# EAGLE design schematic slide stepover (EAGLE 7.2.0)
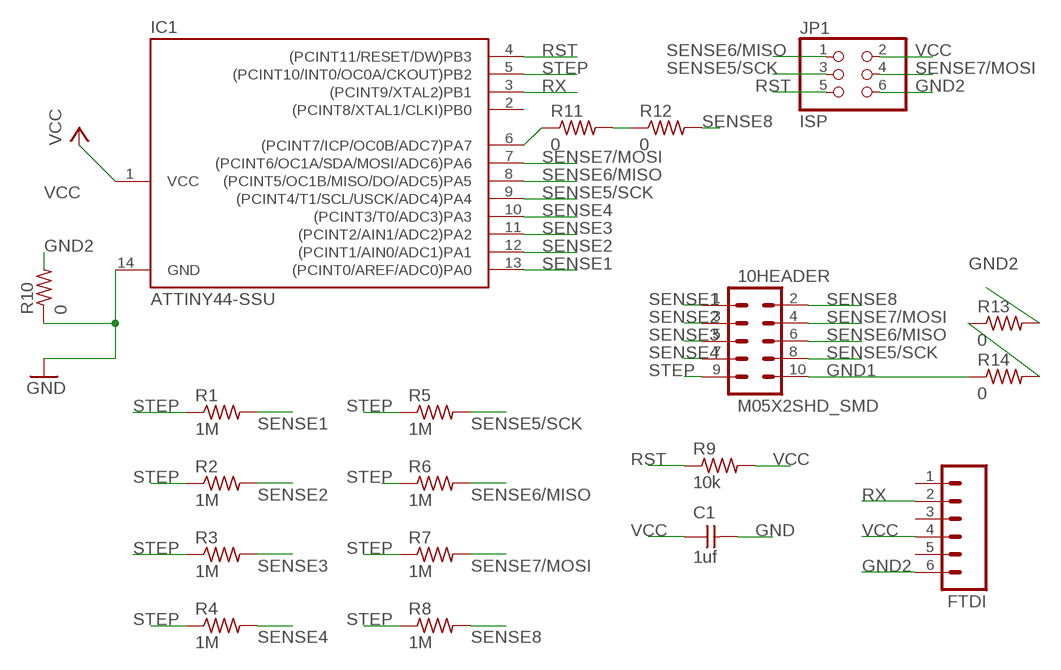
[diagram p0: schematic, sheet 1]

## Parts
10HEADER  M05X2SHD_SMD  [2X5-SHROUDED_SMD]
C1  1uf  UNPOLARIZED_CAPACITOR1206  [1206]
FTDI  M06SMD  [1X06-SMD]
IC1  ATTINY44-SSU  [SOIC14]
JP1  ISP  PINHD-2X3-SMD  [2X03SMD]
R1  1M  RESISTOR1206  [1206]
R2  1M  RESISTOR1206  [1206]
R3  1M  RESISTOR1206  [1206]
R4  1M  RESISTOR1206  [1206]
R5  1M  RESISTOR1206  [1206]
R6  1M  RESISTOR1206  [1206]
R7  1M  RESISTOR1206  [1206]
R8  1M  RESISTOR1206  [1206]
R9  10k  RESISTOR1206  [1206]
R10  0  RESISTOR1206  [1206]
R11  0  RESISTOR1206  [1206]
R12  0  RESISTOR1206  [1206]
R13  0  RESISTOR1206  [1206]
R14  0  RESISTOR1206  [1206]

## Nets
GND: C1.2 IC1.14(GND) R10.1
GND1: 10HEADER.10 R14.1
GND2: FTDI.6 JP1.6 R10.2 R13.2
N$1: R11.2 R12.1
N$2: R13.1 R14.2
N$3: IC1.6((PCINT7/ICP/OC0B/ADC7)PA7) R11.1
RST: IC1.4((PCINT11/RESET/DW)PB3) JP1.5 R9.1
RX: FTDI.2 IC1.3((PCINT9/XTAL2)PB1)
SENSE1: 10HEADER.1 IC1.13((PCINT0/AREF/ADC0)PA0) R1.2
SENSE2: 10HEADER.3 IC1.12((PCINT1/AIN0/ADC1)PA1) R2.2
SENSE3: 10HEADER.5 IC1.11((PCINT2/AIN1/ADC2)PA2) R3.2
SENSE4: 10HEADER.7 IC1.10((PCINT3/T0/ADC3)PA3) R4.2
SENSE5/SCK: 10HEADER.8 IC1.9((PCINT4/T1/SCL/USCK/ADC4)PA4) JP1.3 R5.2
SENSE6/MISO: 10HEADER.6 IC1.8((PCINT5/OC1B/MISO/DO/ADC5)PA5) JP1.1 R6.2
SENSE7/MOSI: 10HEADER.4 IC1.7((PCINT6/OC1A/SDA/MOSI/ADC6)PA6) JP1.4 R7.2
SENSE8: 10HEADER.2 R8.2 R12.2
STEP: 10HEADER.9 IC1.5((PCINT10/INT0/OC0A/CKOUT)PB2) R1.1 R2.1 R3.1 R4.1 R5.1 R6.1 R7.1 R8.1
VCC: C1.1 FTDI.4 IC1.1(VCC) JP1.2 R9.2
Unconnected: FTDI.1 FTDI.3 FTDI.5 IC1.2((PCINT8/XTAL1/CLKI)PB0)

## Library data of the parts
10HEADER = 01_SparkFun:M05X2: Header 5x2 Standard 10-pin dual row 0.1" header. Commonly used with AVR-ISP. Use with Spark Fun Electronics SKU: PRT-00778
C1 = 01_ng:UNPOLARIZED_CAPACITOR: unpolarized_capacitor
FTDI = 01_SparkFun:M06: Header 6 Standard 6-pin 0.1" header. Use with straight break away headers (SKU : PRT-00116), right angle break away headers (PRT-00553), swiss pins (PRT-00743), machine pins (PRT-00117), and female headers (PRT-00115). Molex polarized connector foot print use with SKU : PRT-08094 with associated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
IC1 = 01_fab:ATTINY44
JP1 = 01_fab:PINHD-2X3-SMD: PIN HEADER
R1-R14 = 01_ng:RESISTOR

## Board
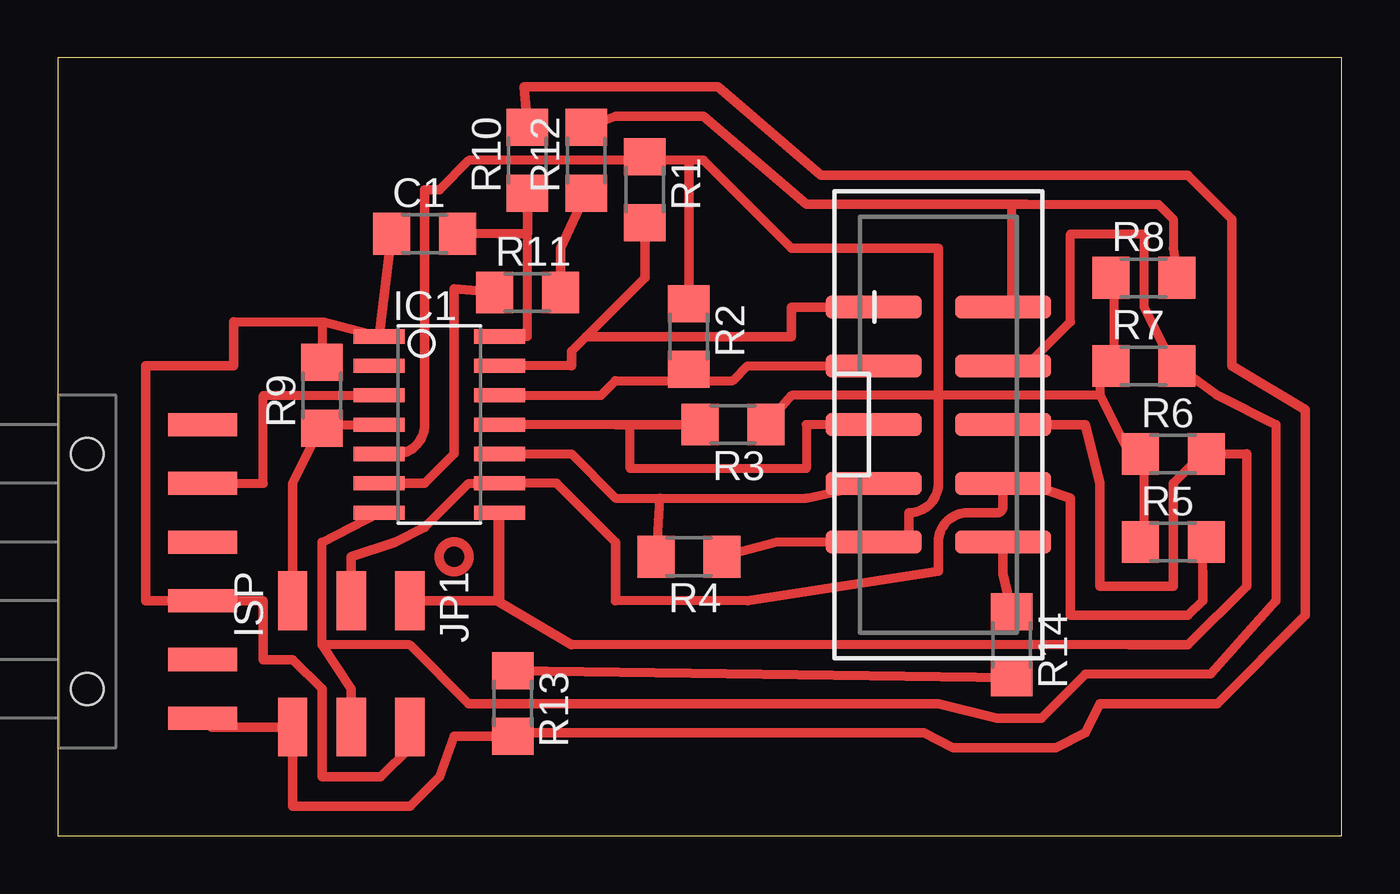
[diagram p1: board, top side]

Size 55.55 x 33.64 mm. Coordinates in mm from the lower left corner, seen from the top.
Outline: 0,0 55.55,0 55.55,33.64 0,33.64 0,0
Copper layers (1*16): Top 0.035mm / dielectric 1.5mm / Bottom 0.035mm
Design rules "default *": minimum track width 0.4mm, minimum drill 0.8mm, track to track 0.4mm, track to pad 0.4mm, pad to pad 0.4mm, via to via 0.4mm, smd to smd 8mil, copper to edge 0mil, drill to drill 0.8mm, minimum pad ring 10mil, minimum via ring 8mil, stop-mask expansion 4mil, vias tented up to drill 0mil, thermal gap 10mil

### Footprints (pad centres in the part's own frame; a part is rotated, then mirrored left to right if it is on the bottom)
2X5-SHROUDED_SMD = smd 4.15 x 1: 1 -2.794,5.08; 2 2.794,5.08; 3 -2.794,2.54; 4 2.794,2.54; 5 -2.794,0; 6 2.794,0; 7 -2.794,-2.54; 8 2.794,-2.54; 9 -2.794,-5.08; 10 2.794,-5.08
1206 = smd 1.6 x 1.803: 1 -1.422,0; 2 1.422,0
1X06-SMD = smd 1 x 3: 1 -6.35,5; 2 -3.81,5; 3 -1.27,5; 4 1.27,5; 5 3.81,5; 6 6.35,5 | hole 1.4: -5.08,0; 5.08,0
SOIC14 = smd 0.61 x 2.21: 1 -3.81,-2.603; 2 -2.54,-2.603; 3 -1.27,-2.603; 4 0,-2.603; 5 1.27,-2.603; 6 2.54,-2.603; 7 3.81,-2.603; 8 3.81,2.603; 9 2.54,2.603; 10 1.27,2.603; 11 0,2.603; 12 -1.27,2.603; 13 -2.54,2.603; 14 -3.81,2.603
2X03SMD = smd 2.54 x 1.27: 1 -2.54,2.54; 2 2.92,2.54; 3 -2.54,0; 4 2.92,0; 5 -2.54,-2.54; 6 2.92,-2.54

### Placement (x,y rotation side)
10HEADER  38.1,17.78 0 top
C1  15.88,26.04 0 top
FTDI  1.27,11.43 270 top
IC1  16.51,17.78 270 top
JP1  12.7,7.62 270 top
R1  25.4,27.94 270 top
R2  27.3,21.59 270 top
R3  29.21,17.78 180 top
R4  27.3,12.07 180 top
R5  48.26,12.7 0 top
R6  48.26,16.51 0 top
R7  46.99,20.32 0 top
R8  46.99,24.13 0 top
R9  11.43,19.05 90 top
R10  20.32,29.21 90 top
R11  20.32,23.5 0 top
R12  22.86,29.21 90 top
R13  19.68,5.71 270 top
R14  41.27,8.26 270 top

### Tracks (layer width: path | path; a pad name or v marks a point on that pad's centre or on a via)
GND
  Top 0.4: 20.32,26.04 20.32,21.59 IC1.14 | 19.05,26.04 C1.2
  Top 0.406: 19.05,26.04 20.32,26.04 R10.1
GND1
  Top 0.406: 10HEADER.10 40.89,11.33 R14.1
GND2
  Top 0.406: FTDI.6 6.65,4.7 JP1.6 10.16,1.27 15.24,1.27 16.51,2.54 17.14,4.29 R13.2 20.32,4.45 37.46,4.45 38.73,3.81 43.18,3.81 44.45,4.45 45.08,5.71 50.16,5.71 53.97,9.53 53.97,18.41 50.8,20.32 50.8,26.67 48.89,28.57 33.02,28.57 28.57,32.38 20.17,32.38 R10.2
N$1
  Top 0.406: R11.2 21.74,25.4 R12.1
N$2
  Top 0.406: R13.1 R14.2
N$3
  Top 0.406: R11.1 17.14,23.65 17.14,16.51 15.88,15.24 IC1.6
RST
  Top 0.4: 10.16,15.24 11.43,17.78 | 11.43,17.78 R9.1 | 11.43,17.78 IC1.4
  Top 0.406: 10.16,15.24 JP1.5
RX
  Top 0.4: IC1.3 8.89,19.05 8.89,15.24 FTDI.2
SENSE1
  Top 0.4: 34.92,22.86 10HEADER.1 | 22.23,20.32 IC1.13 | 25.4,26.67 R1.2
  Top 0.406: 22.86,21.59 31.75,21.59 31.75,22.86 10HEADER.1 | R1.2 25.4,24.13 22.86,21.59 | 22.23,20.32 22.23,20.96 22.86,21.59
SENSE2
  Top 0.4: IC1.12 23.5,19.05 24.13,19.68 27.94,19.68 29.21,19.68 29.84,20.32 10HEADER.3
  Top 0.406: R2.2 27.94,19.68
SENSE3
  Top 0.4: 10HEADER.5 32.38,17.78 32.38,15.88 24.77,15.88 24.77,17.78 24.13,17.78 IC1.11
  Top 0.406: R3.2 24.13,17.78
SENSE4
  Top 0.4: IC1.10 22.23,16.51 24.13,14.61 26.04,14.61 | 26.04,14.61 R4.2 | 10HEADER.7 32.38,14.61 26.04,14.61
SENSE5/SCK
  Top 0.4: 15.88,13.34 17.78,15.24 IC1.9 21.59,15.24 | 49.53,11.43 49.53,12.7 R5.2 | 10HEADER.8 41.91,15.24 | 29.84,10.16 24.13,10.16
  Top 0.406: 29.84,10.16 38.1,11.43 38.1,12.7 arc-90 39.37,13.97 40.64,13.97 arc90 40.89,14.22 10HEADER.8 | 49.53,11.43 49.53,10.16 48.89,9.53 43.81,9.53 43.81,14.61 41.91,15.24 | JP1.3 12.7,12.07 14.61,12.7 15.88,13.34 | 24.13,10.16 24.13,12.7 21.59,15.24
SENSE6/MISO
  Top 0.4: 19.05,10.16 19.05,13.97 IC1.8 | 48.26,15.24 49.53,16.51 R6.2 51.43,16.51 | 10HEADER.6 41.91,17.78 | 46.35,8.26 22.23,8.26
  Top 0.406: JP1.1 19.05,10.16 | IC1.8 19.11,10.1 22.23,8.26 | 46.35,8.26 48.89,8.26 51.43,10.79 51.43,16.51 | 41.91,17.78 44.45,17.78 45.08,15.24 45.08,10.79 48.26,10.79 48.26,15.24
SENSE7/MOSI
  Top 0.4: 12.7,6.35 11.43,8.26 | 11.43,8.26 11.43,12.7 IC1.7 | 10HEADER.4 41.91,20.32 43.81,22.23 43.81,26.04 46.99,26.04 46.99,22.86 48.26,20.32 R7.2 | 11.43,8.26 15.24,8.26 17.78,5.71 | 49.89,7.02 52.7,10.16 52.7,17.78
  Top 0.406: JP1.4 12.7,6.35 | 17.78,5.71 38.1,5.71 40.64,5.08 42.54,5.08 44.45,6.99 49.89,7.02 | 52.7,17.78 50.16,19.05 R7.2
SENSE8
  Top 0.4: R8.2 48.26,25.4 48.26,26.67 47.62,27.3 41.91,27.3 41.27,27.3 41.27,22.86 10HEADER.2
  Top 0.406: 10HEADER.2 40.64,22.86 | R12.2 24.13,31.11 27.94,31.11 32.38,27.3 41.91,27.3
STEP
  Top 0.4: 10HEADER.9 31.11,12.7 R4.1 | R5.1 46.99,12.7 46.99,16.51 R6.1 46.35,16.51 45.08,19.05 | 45.08,19.05 38.1,19.05 31.75,19.05 R3.1 | 45.08,19.05 45.08,20.32 R7.1 45.72,20.32 45.72,24.13 R8.1 | 27.94,22.86 R2.1 | 27.94,29.21 27.3,29.21 25.4,29.21 | 16.51,27.94 17.78,29.21 25.4,29.21 | 25.4,29.21 R1.1
  Top 0.406: 10HEADER.9 36.83,12.7 36.83,13.97 arc90 38.1,15.24 38.1,19.05 38.1,25.4 31.75,25.4 27.94,29.21 | 27.94,22.86 27.3,23.5 27.3,29.21 | 16.51,27.94 15.88,27.94 15.88,17.78 arc-90 14.61,16.51 IC1.5
VCC
  Top 0.4: 11.43,22.23 IC1.1 13.97,21.59 | 5.71,10.16 FTDI.4 | 7.62,22.23 11.43,22.23 | 11.43,22.23 R9.2
  Top 0.406: 7.62,22.23 7.62,20.32 3.81,20.32 3.81,10.16 5.71,10.16 | JP1.2 15.24,3.81 13.97,2.54 11.43,2.54 11.43,6.35 10.16,7.62 8.89,7.62 8.89,10.16 FTDI.4 | C1.1 IC1.1
(copper drawn outside any net)
  shapes: Top circle x1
